(* Logix 5000 DataType export Yaskawa_OUT_to_Servo; software revision 17.00 *)

TYPE Yaskawa_OUT_to_Servo :   // Structure of data sent out to the Yaskawa SigmaLogic controller v2.4.0
STRUCT
   b00_ServoOn : BOOL;   // Servo On
   b01_Stop : BOOL;   // Stops All Current Motion in Progress
   b02_Home : BOOL;   // Start Homing Process
   b03_MoveStart1 : BOOL;   // Start Current Motion
   b06_SuperImpose : BOOL;
   b07_ServoAlarmReset : BOOL;   // Servo Alarm Reset
   b08_ControllerAlarmReset : BOOL;   // SigmaLogic Alarm Reset
   b09_MoveStart2 : BOOL;   // Start Second Motion (Blended Move)
   b10_MoveAbort : BOOL;   // Abort Current Move
   b11_MovePause : BOOL;   // Pause Current Move
   b12_SeqPause : BOOL;   // Indexing Sequence Pause
   b13_SeqResume : BOOL;   // Indexing Sequence Resume
   b14_SeqCancel : BOOL;   // Indexing Sequence Cancel
   b15_AbsEncoderReset : BOOL;   // Absolute Encoder Reset
   b16_SeqStart : BOOL;   // Start Indexing Sequence
   b17_SeqEditSpeed : BOOL;   // Enter Edit Speed
   b18_SeqEditDistance : BOOL;   // Enter Distance Edit
   b19_PLSEnable : BOOL;   // Enable PLS execution
   b20_PLSActivateOutput1 : BOOL;   // Activate PLS output1 switch logic
   b21_PLSActivateOutput2 : BOOL;   // Activate PLS output2 switch logic
   b22_PLSActivateOutput3 : BOOL;   // Activate PLS output3 switch logic
   b23_PLSActivateOutput4 : BOOL;   // Activate PLS output4 switch logic
   b24_SetClock : BOOL;   // Set the remote controller clock with data provided by the PLC
   RebootController : BOOL;
   UseExternalEncoder : BOOL;   // Use External Encoder when executing MAHSP_Yaskawa
   b32_HeatbeatAnswer : BOOL;   // Heartbeat Answer
   BrakeBypassRequest : BOOL;
   SetFwdTorqueLimit : BOOL;
   SetRevTorqueLimit : BOOL;
   TorqueLimit : DINT;
   TorqueRamp : DINT;
   HomeMethod : INT;
   HomeSpeed : DINT;
   HomeAccDec : DINT;   // Home Move Acceleration/Deceleration Rate
   HomeBackOffDistance : DINT;
   HomeCreepSpeed : DINT;
   HomeCreepDistanceLimit : DINT;
   HomeCreepTimeLimit : DINT;
   HomeOffsetDistance : DINT;
   HomeOffsetSpeed : DINT;
   HomePostion : DINT;
   HomeTorque : DINT;
   HomeInputNo : DINT;
   HomeApproachTimeLimit : DINT;
   HomeApproachDistLimit : DINT;
   HomeDirection : INT;
   HomeSwitchMode : INT;
   MoveType : INT;
   MoveDirection : INT;
   MoveAccel1 : DINT;
   MoveAccel2 : DINT;
   MoveDecel1 : DINT;
   MoveDecel2 : DINT;
   MoveSpeed1 : DINT;
   MoveSpeed2 : DINT;
   MoveDistance1 : DINT;
   MoveDistance2 : DINT;
   MovePosition1 : DINT;
   MovePosition2 : DINT;
   RegistrationDistance : DINT;
   GearNumerator : DINT;
   GearDenominator : DINT;
   SuperImposeDistance : DINT;
   Resolution : INT;
   RegistrationDirection : INT;
   TuningLevel : INT;
   SequenceStep : INT;   // Staring Sequence Step Number
   SequenceEditStep : INT;   // Sequence Step Number to Edit
   FlagCommandBits1 : DINT;   // Flag Commands. 1..64 are General Flags, Bits 0..31 correspond to Flag 1..32
   FlagCommandBits2 : DINT;   // Flag Commands cont. 1..64 are General Flags, Bits 0..31 correspond to Flag 33..64
   DigitalOutCommandBits : DINT;   // Digital Output commands. Bits 0-7 correspond to CN13 Digital Outputs 0-7, used as Flag 73-80. Bits 8-10 correspond to CN1 Digital Outputs 0-2 used as Flag 88-90"
   SequenceEditSpeed : DINT;
   SequenceEditDistance : DINT;
   FeedRateOverride : INT;
   HSI_Enable : BOOL;
   HSI_MoveMode : BOOL;   // 0=Relative; 1=Moves per Cycle
   HSI_CalcMethod : BOOL;   // 0=Accel/Decel; 1=Time
   HSI_MoveDirection : BOOL;   // 0 = Negative; 1 = Positive
   HSI_TriggerFlag : INT;
   HSI_MovingFlag : INT;
   HSI_DwellingFlag : INT;
   HSI_DoneFlag : INT;
   HSI_MoveType : INT;   // 0=Single; 1=Repeat; 2=Repeat "x" times
   HSI_RepeatNumber : INT;
   HSI_Distance : DINT;
   HSI_Speed : DINT;
   HSI_Accel : DINT;
   HSI_MoveTime : DINT;
   HSI_DwellTime : DINT;
   PLS_OutputFlag1 : INT;
   PLS_OutputFlag2 : INT;
   PLS_OutputFlag3 : INT;
   PLS_OutputFlag4 : INT;
   PLS_OnPosition1 : DINT;
   PLS_OffPosition1 : DINT;
   PLS_OnPosition2 : DINT;
   PLS_OffPosition2 : DINT;
   PLS_OnPosition3 : DINT;
   PLS_OffPosition3 : DINT;
   PLS_OnPosition4 : DINT;
   PLS_OffPosition4 : DINT;
   PLS_OnCompensation1 : INT;
   PLS_OffCompensation1 : INT;
   PLS_OnCompensation2 : INT;
   PLS_OffCompensation2 : INT;
   PLS_OnCompensation3 : INT;
   PLS_OffCompensation3 : INT;
   PLS_OnCompensation4 : INT;
   PLS_OffCompensation4 : INT;
   RTC_Year : INT;
   RTC_Month : INT;
   RTC_Day : INT;
   RTC_Hour : INT;
   RTC_Min : INT;
   RTC_Sec : INT;
   StopDecel : DINT;
   AnalogOutput : INT;   // CN13, AO_01 [mV]
END_STRUCT
END_TYPE
